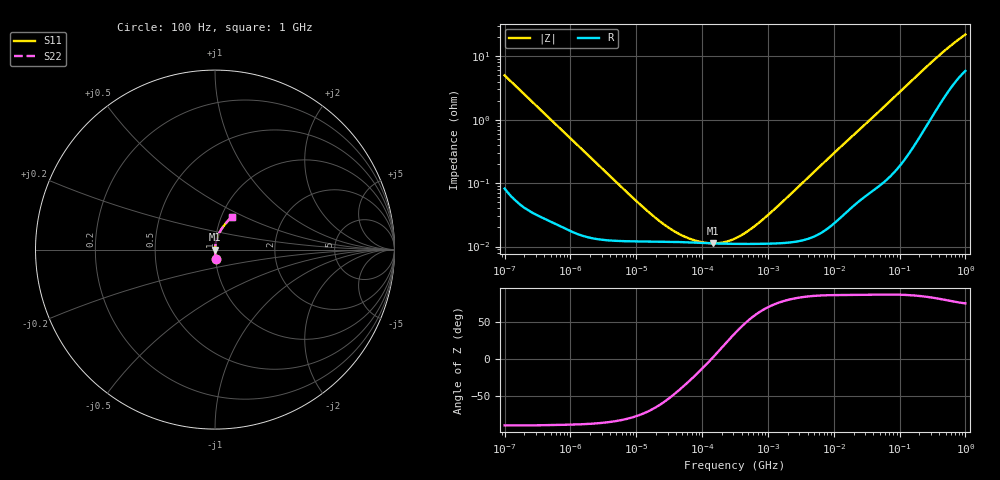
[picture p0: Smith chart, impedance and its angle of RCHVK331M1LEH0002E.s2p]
! RCHVK331M1LEH0002E  S-PARAMETER MODEL  (AEC-Q200 qualified)
! Model Generated by ELNA Corporation (http://www.ty-top.com)
! Version 1.0
! ELNA Control No. 201216
! Copyright (c) 2020 ELNA CO.,LTD. All Rights Reserved.
! Products Name : CONDUCTIVE POLYMER HYBRID ALUMINUM ELECTROLYTIC CAPACITORS
! Characteristics :
!  Capacitance  :  330uF  ,  Rated voltage  :  10V
!  Operating Temp. Range  :  -55 to +125 degC  ,  Endurance  :  4000hr at 125 degC
!  Dimension D  :  8mm  ,  Dimension L  :  10mm
! Frequency Range : 100Hz - 1GHz
! External Node Assignments :
!  1  o---| |---o  2
# MHz S RI R 50
!Freq[MHz].  S11 Real  S11 Imag  S21 Real  S21 Imag  S12 Real  S12 Imag  S22 Real  S22 Imag
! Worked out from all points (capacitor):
!   401 points, 100 Hz to 1 GHz, reference 50 ohm
!   read as one part in series: C = 318 uF near 108 Hz
!   lowest |Z| = 11.2 mohm at 147.1 kHz (marker M1)
!   series resonance near 138.9 kHz, so ESL is about 4.1 nH
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0.0001  0.00332 -0.0499  0.9967 0.0499  0.9967 0.0499  0.00332 -0.0499
0.000113  0.00267 -0.0442  0.9973 0.0442  0.9973 0.0442  0.00267 -0.0442
0.000285  0.000638 -0.0176  0.9994 0.0176  0.9994 0.0176  0.000638 -0.0176
0.001488  0.000161 -0.00343  0.9998 0.00343  0.9998 0.00343  0.000161 -0.00343
0.00912  0.000121 -0.000559  0.9999 0.000559  0.9999 0.000559  0.000121 -0.000559
0.014791  0.00012 -0.000343  0.9999 0.000343  0.9999 0.000343  0.00012 -0.000343
0.022131  0.00012 -0.000227  0.9999 0.000227  0.9999 0.000227  0.00012 -0.000227
0.035892  0.000119 -0.000135  0.9999 0.000135  0.9999 0.000135  0.000119 -0.000135
0.05821  0.000117 -7.53e-05  0.9999 7.53e-05  0.9999 7.53e-05  0.000117 -7.53e-05
0.094406  0.000114 -3.12e-05  0.9999 3.12e-05  0.9999 3.12e-05  0.000114 -3.12e-05
0.147062  0.000112 4.6e-06  0.9999 -4.6e-06  0.9999 -4.6e-06  0.000112 4.6e-06
0.220039  0.000111 3.9e-05  0.9999 -3.9e-05  0.9999 -3.9e-05  0.000111 3.9e-05
0.316228  0.00011 7.58e-05  0.9999 -7.58e-05  0.9999 -7.58e-05  0.00011 7.58e-05
0.492606  0.00011 0.000135  0.9999 -0.000135  0.9999 -0.000135  0.00011 0.000135
0.798914  0.000111 0.000232  0.9999 -0.000232  0.9999 -0.000232  0.000111 0.000232
1.522299  0.000113 0.000452  0.9999 -0.000452  0.9999 -0.000452  0.000113 0.000452
4.704354  0.000142 0.0014  0.9999 -0.0014  0.9999 -0.0014  0.000142 0.0014
69.9842  0.0016 0.0191  0.9984 -0.0191  0.9984 -0.0191  0.0016 0.0191
176.8072  0.00647 0.0469  0.9935 -0.0469  0.9935 -0.0469  0.00647 0.0469
380.1894  0.0243 0.0937  0.9757 -0.0937  0.9757 -0.0937  0.0243 0.0937
668.3439  0.0571 0.1429  0.9429 -0.1429  0.9429 -0.1429  0.0571 0.1429
1000  0.0922 0.1823  0.9078 -0.1823  0.9078 -0.1823  0.0922 0.1823
